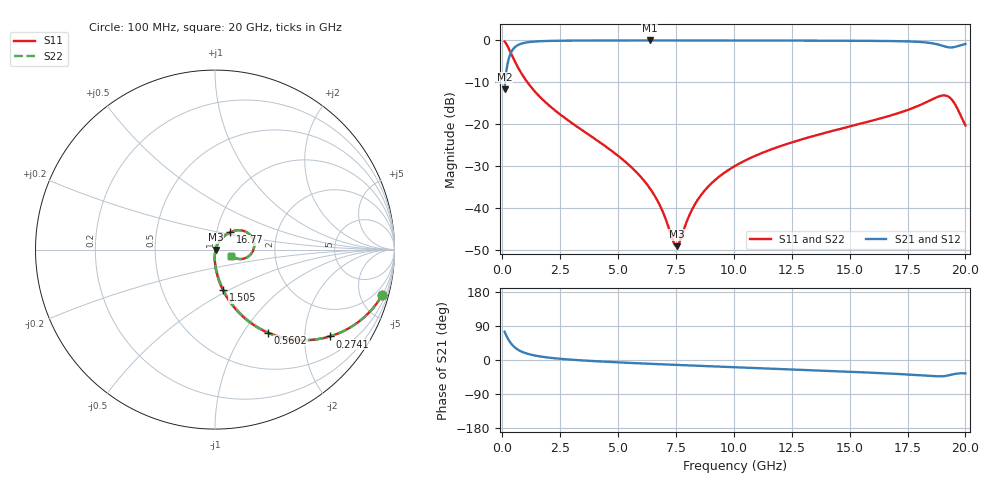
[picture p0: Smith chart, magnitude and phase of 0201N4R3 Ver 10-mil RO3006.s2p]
# GHz S MA R 50
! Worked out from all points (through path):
!   1601 points, 100 MHz to 20 GHz, reference 50 ohm
!   highest |S21| = -0.03 dB at 6.369 GHz (marker M1); lowest = -11.7 dB at 100 MHz (marker M2)
!   group delay of S21, straight-line fit = 8.5 ps
!   lowest |S11| = -49.0 dB at 7.525 GHz (marker M3), VSWR 1.01, Z = 50.3 - j0.0793 ohm
!   |S11| at or under -10 dB: 1.085 GHz to end of sweep
!   |S22| runs from -49.0 to -0.3 dB; largest |S21 - S12| = 0
!   S11 on the Smith chart (normalised r, x): 100 MHz: 0.98, -7.31; 274.1 MHz: 0.98, -2.66; 560.2 MHz: 0.98, -1.30; 1.505 GHz: 0.98, -0.47; 16.77 GHz: 1.16, +0.23; 20 GHz: 1.20, -0.08
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0.1  0.9652 -15.3  0.2612 74.7  0.2612 74.7  0.9652 -15.3
0.274125  0.8025 -37.1  0.596 52.9  0.596 52.9  0.8025 -37.1
0.5601875  0.5481 -57.6  0.8353 32.3  0.8353 32.3  0.5481 -57.6
0.920875  0.3674 -69.8  0.9287 20.0  0.9287 20.0  0.3674 -69.8
1.505437  0.2294 -78.9  0.9716 10.7  0.9716 10.7  0.2294 -78.9
3.420812  0.08614 -89.3  0.9937 -1.0  0.9937 -1.0  0.08614 -89.3
5.286437  0.03633 -92.3  0.9962 -7.1  0.9962 -7.1  0.03633 -92.3
6.3685  0.01735 -89.2  0.9964 -10.0  0.9964 -10.0  0.01735 -89.2
6.741625  0.01174 -84.4  0.9964 -11.0  0.9964 -11.0  0.01174 -84.4
7.388375  0.00398 -40.9  0.9963 -12.6  0.9963 -12.6  0.00398 -40.9
7.525188  0.003538 -12.9  0.9963 -13.0  0.9963 -13.0  0.003538 -12.9
8.1595  0.009222 51.9  0.9961 -14.6  0.9961 -14.6  0.009222 51.9
8.569937  0.0142 59.0  0.9959 -15.6  0.9959 -15.6  0.0142 59.0
9.20425  0.02188 62.5  0.9956 -17.1  0.9956 -17.1  0.02188 62.5
10.05  0.03191 63.4  0.9951 -19.1  0.9951 -19.1  0.03191 63.4
13.37081  0.07164 58.7  0.9918 -27.0  0.9918 -27.0  0.07164 58.7
16.69162  0.1254 49.4  0.9808 -35.6  0.9808 -35.6  0.1254 49.4
16.76625  0.1272 49.0  0.9802 -35.9  0.9802 -35.9  0.1272 49.0
18.43287  0.1901 33.3  0.934 -41.9  0.934 -41.9  0.1901 33.3
19.11694  0.2207 8.2  0.8446 -42.3  0.8446 -42.3  0.2207 8.2
19.47762  0.1867 -12.6  0.8271 -37.6  0.8271 -37.6  0.1867 -12.6
20  0.09678 -20.4  0.9057 -35.3  0.9057 -35.3  0.09678 -20.4
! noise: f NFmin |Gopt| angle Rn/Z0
0.1  0.0006382  0.9338  0.6789  0.002145
2.301  0.004329  0.7888  4.221  0.004216
4.515  0.007038  0.7508  7.935  0.005666
6.729  0.009442  0.7274  11.65  0.00682
8.943  0.01172  0.7118  15.34  0.007878
11.14  0.01404  0.7027  18.99  0.009012
13.36  0.01678  0.703  22.63  0.01066
15.57  0.02144  0.7267  26.29  0.01481
17.79  0.03988  0.8236  30.09  0.04431
20  0.08804  0.9066  33.89  0.1894
